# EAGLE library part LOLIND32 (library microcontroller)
Wemos Lolin D32 Lolin D32 is a development board based on ESP32. On this schematic, this board is designed with battery port. Pins VP and VN are Not Connected pins.
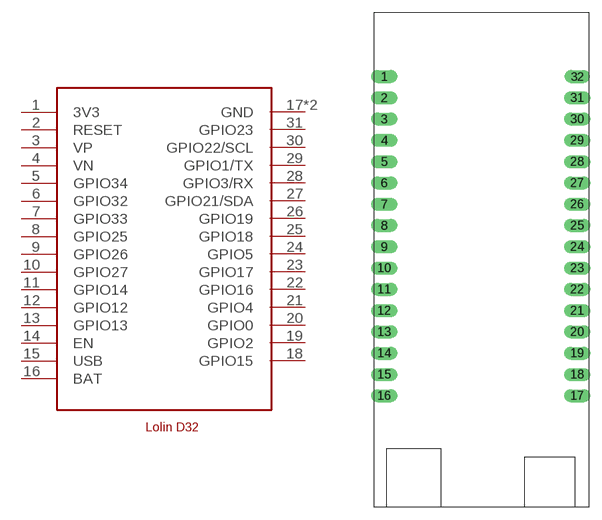
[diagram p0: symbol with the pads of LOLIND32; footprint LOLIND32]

Designator prefix -

## LOLIND32  [LOLIND32]
1  3V3  pwr
2  RESET  in
3  VP  nc
4  VN  nc
5  GPIO34  in
6  GPIO32
7  GPIO33
8  GPIO25
9  GPIO26
10  GPIO27
11  GPIO14
12  GPIO12
13  GPIO13
14  EN  in
15  USB  pwr
16  BAT  pwr
17  GND  pwr
18  GPIO15
19  GPIO2
20  GPIO0
21  GPIO4
22  GPIO16
23  GPIO17
24  GPIO5
25  GPIO18
26  GPIO19
27  GPIO21/SDA
28  GPIO3/RX
29  GPIO1/TX
30  GPIO22/SCL
31  GPIO23
32  GND  pwr

## Footprint LOLIND32 (pad centres in mm)
Wemos Lolin D32 ESP32 development board with battery port. VP and VN are Not Connected pins
drill 1 pad 1.575 long: 1 -11.43,21.59; 2 -11.43,19.05; 3 -11.43,16.51; 4 -11.43,13.97; 5 -11.43,11.43; 6 -11.43,8.89; 7 -11.43,6.35; 8 -11.43,3.81; 9 -11.43,1.27; 10 -11.43,-1.27; 11 -11.43,-3.81; 12 -11.43,-6.35; 13 -11.43,-8.89; 14 -11.43,-11.43; 15 -11.43,-13.97; 16 -11.43,-16.51; 17 11.58,-16.51; 18 11.58,-13.97; 19 11.58,-11.43; 20 11.58,-8.89; 21 11.58,-6.35; 22 11.58,-3.81; 23 11.58,-1.27; 24 11.58,1.27; 25 11.58,3.81; 26 11.58,6.35; 27 11.58,8.89; 28 11.58,11.43; 29 11.58,13.97; 30 11.58,16.51; 31 11.58,19.05
drill 1 pad 1.524 long: 32 11.58,21.59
